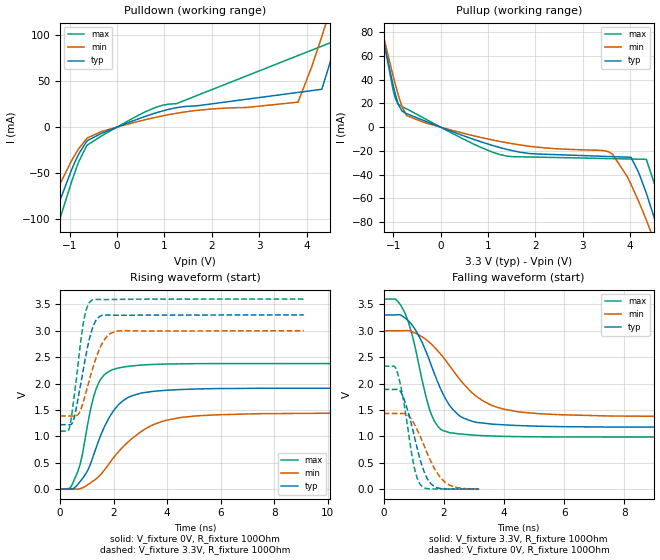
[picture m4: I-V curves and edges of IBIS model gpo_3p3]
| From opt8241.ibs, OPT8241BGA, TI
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|   gpo_3p3 Model
[Model]   gpo_3p3
Model_type   Output
Polarity   Non-Inverting
Vmeas = 1.65
Vref = 0
Cref = 2pF
Rref = 150
|   typ   min   max
|   (nom PVT)   (fast PVT)   (slow PVT)
C_comp   2.070e-12   1.832e-12   2.328e-12
| Where nom  PVT is Nominal Process, 3.3V, 27C
|   Fast PVT is Strong Process,  3.6V, -40C
|   Slow PVT is Weak Process,   3V, 125C
[Voltage Range]   3.3   3   3.6
|Junction Temperature
[Temperature Range]   27   125   -40
[Pullup Reference]   3.3   3   3.6
[Pulldown Reference]   0   0   0
[Power Clamp Reference]   3.3   3   3.6
[GND Clamp Reference]   0   0   0
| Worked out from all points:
|   slope of the pulldown table from 0 to 0.495 V, typ, clamps not added: 50.4 ohm
|   slope of the pullup table from 0 to 0.495 V, typ, clamps not added: 66.5 ohm
|   falling waveform, V_fixture 3.3V, R_fixture 100Ohm: 20-80 % time 954ps typ, 1.51ns min, 628ps max; typ from 3.3 V to 1.22 V
|   rising waveform, V_fixture 0V, R_fixture 100Ohm: 20-80 % time 990ps typ, 1.67ns min, 583ps max; typ from 0 V to 1.89 V
|   rising waveform, V_fixture 3.3V, R_fixture 100Ohm: 20-80 % time 475ps typ, 594ps min, 372ps max; typ from 1.22 V to 3.3 V
|   falling waveform, V_fixture 0V, R_fixture 100Ohm: 20-80 % time 527ps typ, 706ps min, 398ps max; typ from 1.89 V to 0.002 V
[Pulldown]
|   Voltage   I(typ)   I(min)   I(max)
-3.3V     -1.18A     -1.018A    -1.312A
-1.657V   -155.1mA   -111.6mA   -216.9mA
-1.457V   -114.3mA   -88.18mA   -141.2mA
-871.2mV  -36mA      -28.68mA   -46.33mA
-625.2mV  -14.68mA   -11.79mA   -19.44mA
1.085V    19.28mA    13.51mA    24.94mA
3.822V    37.76mA    27.19mA    77.85mA
4.323V    41.18mA    98.57mA    88.06mA
4.472V    65.92mA    122.6mA    91.1mA
4.59V     86.49mA    141.6mA    93.49mA
5.095V    178.9mA    223.1mA    123.6mA
6.6V      456.3mA    467mA      444.5mA
[Pullup]
|   Voltage   I(typ)   I(min)   I(max)
-3.3V     461.2mA    422.2mA    515mA
-1.003V   35.59mA    43.43mA    31.53mA
-888mV    18.83mA    26.4mA     19.24mA
-717mV    11.37mA    9.68mA     15.43mA
1.101V    -15.51mA   -10.86mA   -21.15mA
3.546V    -24.77mA   -20.72mA   -26.53mA
4.02V     -25.44mA   -48.23mA   -26.91mA
4.343V    -55.62mA   -78.29mA   -27.18mA
4.584V    -85.58mA   -103.4mA   -56.22mA
4.736V    -106mA     -126.5mA   -79.04mA
4.818V    -117.7mA   -154mA     -92.23mA
6.6V      -1.176A    -1.2A      -1.101A
[Ramp]
R_load = 100
|   typ   min   max
dV/dt_r   1.13322/9.7966e-10   0.859097/1.66391e-09   1.39879/5.7741e-10
dV/dt_f   1.24861/9.48055e-10   0.969562/1.49836e-09   1.50635/6.26169e-10
[Falling Waveform]
V_fixture = 3.3V
V_fixture_min = 3V
V_fixture_max = 3.6V
R_fixture = 100Ohm
|   Time   V(typ)   V(min)   V(max)
0s        3.3V       3V         3.6V
388ps     3.3V       3V         3.6V
698ps     3.248V     3.002V     3.345V
964ps     3.094V     2.975V     2.882V
1.51ns    2.456V     2.785V     1.539V
1.896ns   1.895V     2.555V     1.134V
2.52ns    1.389V     2.084V     1.045V
3.564ns   1.233V     1.593V     1.006V
5.818ns   1.184V     1.41V      988.2mV
1us       1.219V     1.384V     1.089V
[Rising Waveform]
V_fixture = 0V
V_fixture_min = 0V
V_fixture_max = 0V
R_fixture = 100Ohm
|   Time   V(typ)   V(min)   V(max)
0s        771.9pV    32.35nV    444.8pV
372ps     -1.684mV   60.44uV    24.6mV
662ps     88.9mV     -271.4uV   337.5mV
1.25ns    644.9mV    158.5mV    1.746V
1.662ns   1.19V      367mV      2.172V
2.162ns   1.589V     696.8mV    2.292V
2.688ns   1.767V     959.3mV    2.334V
3.55ns    1.855V     1.235V     2.362V
5.044ns   1.896V     1.384V     2.376V
511.3ns   1.892V     1.432V     2.341V
[Rising Waveform]
V_fixture = 3.3V
V_fixture_min = 3V
V_fixture_max = 3.6V
R_fixture = 100Ohm
|   Time   V(typ)   V(min)   V(max)
0s        1.22V      1.384V     1.098V
316ps     1.22V      1.384V     1.118V
484ps     1.28V      1.384V     1.606V
700ps     1.8V       1.43V      2.507V
888ps     2.328V     1.692V     3.205V
1.038ns   2.723V     1.969V     3.487V
1.19ns    3.021V     2.242V     3.581V
1.648ns   3.296V     2.827V     3.59V
2.102ns   3.294V     2.993V     3.594V
9.1ns     3.3V       3V         3.6V
[Falling Waveform]
V_fixture = 0V
V_fixture_min = 0V
V_fixture_max = 0V
R_fixture = 100Ohm
|   Time   V(typ)   V(min)   V(max)
0s        1.888V     1.432V     2.329V
354ps     1.888V     1.432V     2.328V
462ps     1.888V     1.432V     2.195V
690ps     1.679V     1.43V      1.575V
992ps     1.061V     1.258V     477mV
1.222ns   536.5mV    987.5mV    83.22mV
1.432ns   214.7mV    701.2mV    11.29mV
1.584ns   93.77mV    506.6mV    2.919mV
2.054ns   3.034mV    123.6mV    2.97mV
3.176ns   1.652mV    -26.77uV   587.4uV
